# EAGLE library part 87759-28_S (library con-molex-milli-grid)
HEADER
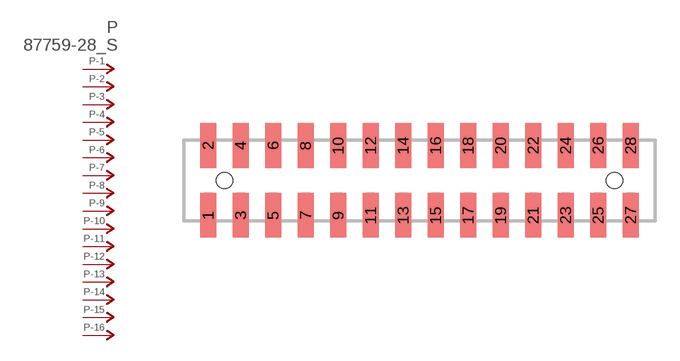
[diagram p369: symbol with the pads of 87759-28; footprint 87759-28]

Designator prefix P; gates -1=P-NV -2=P-N -3=P-N -4=P-N -5=P-N -6=P-N -7=P-N -8=P-N -9=P-N -10=P-N -11=P-N -12=P-N -13=P-N -14=P-N -15=P-N -16=P-N -17=P-N -18=P-N -19=P-N -20=P-N -21=P-N -22=P-N -23=P-N -24=P-N -25=P-N -26=P-N -27=P-N -28=P-N

## 87759-28_S  [87759-28]
1  -1:P  pas
2  -2:P  pas
3  -3:P  pas
4  -4:P  pas
5  -5:P  pas
6  -6:P  pas
7  -7:P  pas
8  -8:P  pas
9  -9:P  pas
10  -10:P  pas
11  -11:P  pas
12  -12:P  pas
13  -13:P  pas
14  -14:P  pas
15  -15:P  pas
16  -16:P  pas
17  -17:P  pas
18  -18:P  pas
19  -19:P  pas
20  -20:P  pas
21  -21:P  pas
22  -22:P  pas
23  -23:P  pas
24  -24:P  pas
25  -25:P  pas
26  -26:P  pas
27  -27:P  pas
28  -28:P  pas

## Footprint 87759-28 (pad centres in mm)
HEADER SMD Dual Row, Vertical
smd 1 x 2.75: 1 -13,-2.15; 2 -13,2.15; 3 -11,-2.15; 4 -11,2.15; 5 -9,-2.15; 6 -9,2.15; 7 -7,-2.15; 8 -7,2.15; 9 -5,-2.15; 10 -5,2.15; 11 -3,-2.15; 12 -3,2.15; 13 -1,-2.15; 14 -1,2.15; 15 1,-2.15; 16 1,2.15; 17 3,-2.15; 18 3,2.15; 19 5,-2.15; 20 5,2.15; 21 7,-2.15; 22 7,2.15; 23 9,-2.15; 24 9,2.15; 25 11,-2.15; 26 11,2.15; 27 13,-2.15; 28 13,2.15
hole 1 at -12,0
hole 1 at 12,0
